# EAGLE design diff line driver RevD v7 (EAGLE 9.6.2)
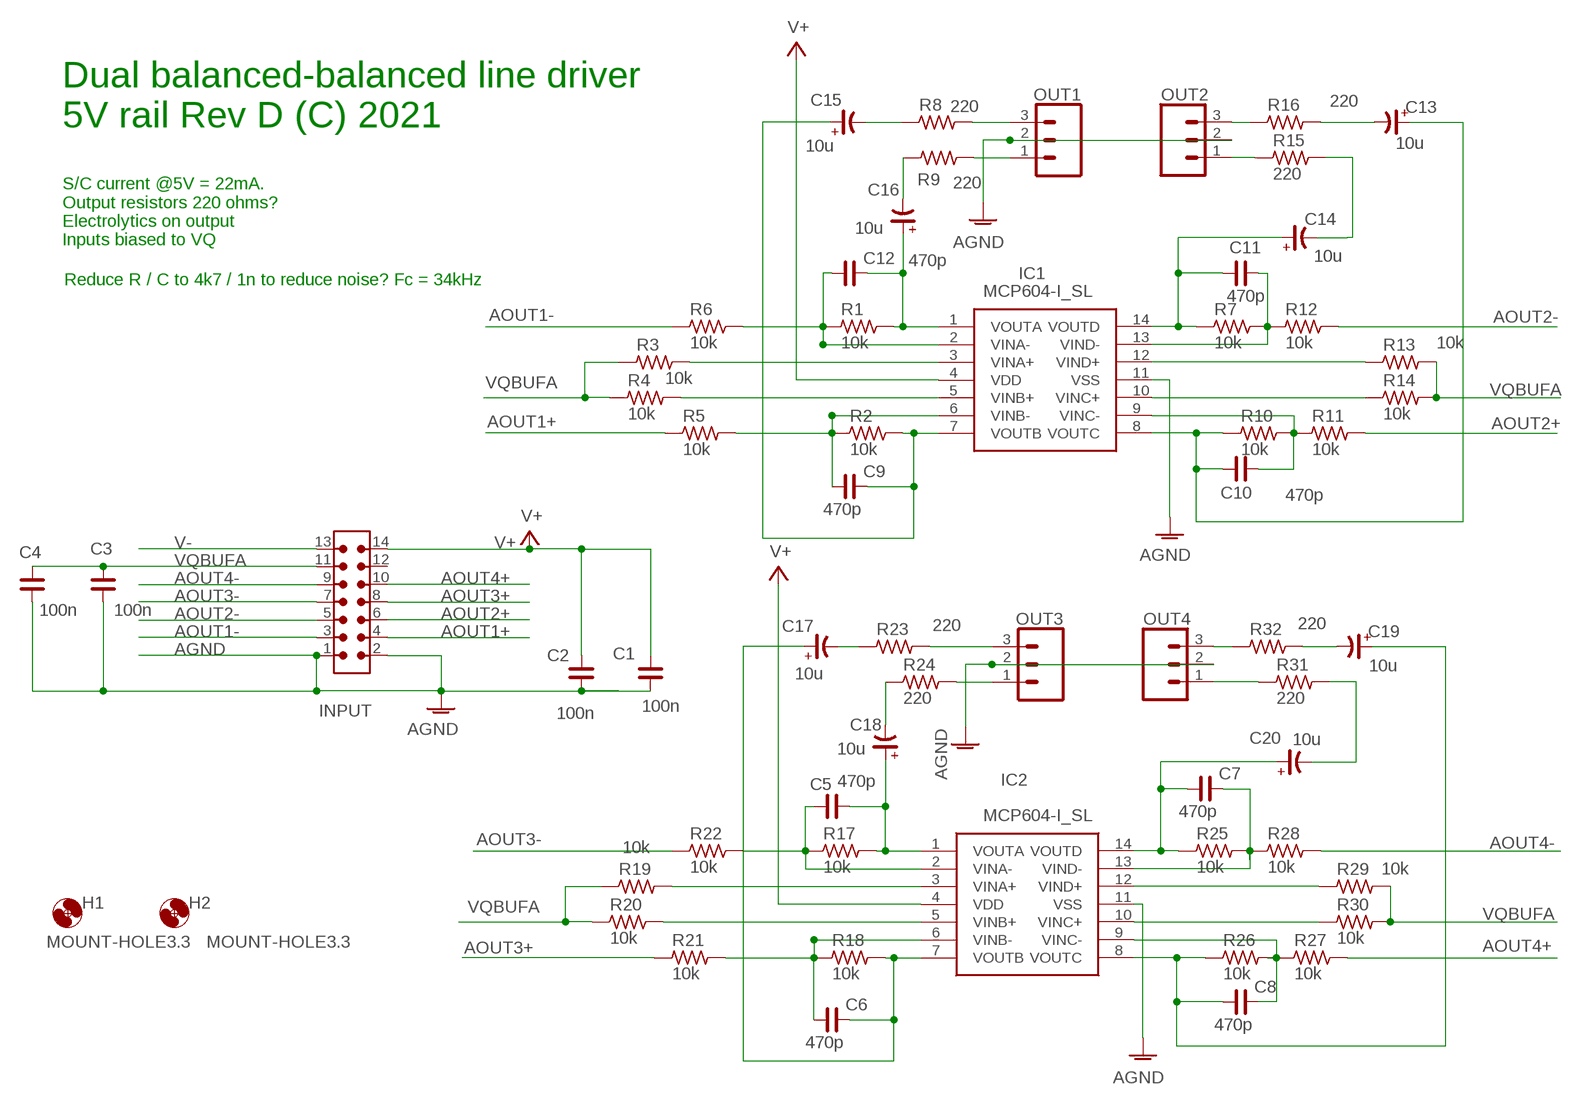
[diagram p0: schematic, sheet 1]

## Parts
C1  100n  C_0805  [C0805]
C2  100n  C_0805  [C0805]
C3  100n  C_0805  [C0805]
C4  100n  C_0805  [C0805]
C5  470p  C_0805  [C0805]
C6  470p  C_0805  [C0805]
C7  470p  C_0805  [C0805]
C8  470p  C_0805  [C0805]
C9  470p  C_0805  [C0805]
C10  470p  C_0805  [C0805]
C11  470p  C_0805  [C0805]
C12  470p  C_0805  [C0805]
C13  10u  CP_SV-C  [CSV-C]
C14  10u  CP_SV-C  [CSV-C]
C15  10u  CP_SV-C  [CSV-C]
C16  10u  CP_SV-C  [CSV-C]
C17  10u  CP_SV-C  [CSV-C]
C18  10u  CP_SV-C  [CSV-C]
C19  10u  CP_SV-C  [CSV-C]
C20  10u  CP_SV-C  [CSV-C]
H1  MOUNT-HOLE3.3  [3,3]
H2  MOUNT-HOLE3.3  [3,3]
IC1  MCP604-I_SL  [SOIC127P600X175-14N]
IC2  MCP604-I_SL  [SOIC127P600X175-14N]
INPUT  6120XX21621_61201421621  [61201421621]
OUT1  CONN_03  [1X03]
OUT2  CONN_03  [1X03]
OUT3  CONN_03  [1X03]
OUT4  CONN_03  [1X03]
R1  10k  R_0805  [R0805]
R2  10k  R_0805  [R0805]
R3  10k  R_0805  [R0805]
R4  10k  R_0805  [R0805]
R5  10k  R_0805  [R0805]
R6  10k  R_0805  [R0805]
R7  10k  R_0805  [R0805]
R8  220  R_0805  [R0805]
R9  220  R_0805  [R0805]
R10  10k  R_0805  [R0805]
R11  10k  R_0805  [R0805]
R12  10k  R_0805  [R0805]
R13  10k  R_0805  [R0805]
R14  10k  R_0805  [R0805]
R15  220  R_0805  [R0805]
R16  220  R_0805  [R0805]
R17  10k  R_0805  [R0805]
R18  10k  R_0805  [R0805]
R19  10k  R_0805  [R0805]
R20  10k  R_0805  [R0805]
R21  10k  R_0805  [R0805]
R22  10k  R_0805  [R0805]
R23  220  R_0805  [R0805]
R24  220  R_0805  [R0805]
R25  10k  R_0805  [R0805]
R26  10k  R_0805  [R0805]
R27  10k  R_0805  [R0805]
R28  10k  R_0805  [R0805]
R29  10k  R_0805  [R0805]
R30  10k  R_0805  [R0805]
R31  220  R_0805  [R0805]
R32  220  R_0805  [R0805]

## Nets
AGND: C1.1 C2.1 C3.1 C4.1 IC1.11(VSS) IC2.11(VSS) INPUT.1 INPUT.2 OUT1.2 OUT2.2 OUT3.2 OUT4.2
AOUT1+: INPUT.4 R5.1
AOUT1-: INPUT.3 R6.1
AOUT2+: INPUT.6 R11.2
AOUT2-: INPUT.5 R12.2
AOUT3+: INPUT.8 R21.1
AOUT3-: INPUT.7 R22.1
AOUT4+: INPUT.10 R27.2
AOUT4-: INPUT.9 R28.2
N$1: C12.1 IC1.2(VINA-) R1.1 R6.2
N$2: C11.1 C14.+ IC1.14(VOUTD) R7.1
N$3: IC1.3(VINA+) R3.2
N$4: C12.2 C16.+ IC1.1(VOUTA) R1.2
N$5: C9.2 C15.+ IC1.7(VOUTB) R2.2
N$6: IC1.5(VINB+) R4.2
N$7: C9.1 IC1.6(VINB-) R2.1 R5.2
N$8: C10.1 C13.+ IC1.8(VOUTC) R10.1
N$9: OUT2.3 R16.1
N$10: OUT2.1 R15.1
N$11: OUT1.3 R8.2
N$12: OUT1.1 R9.2
N$13: C5.2 C18.+ IC2.1(VOUTA) R17.2
N$14: C10.2 IC1.9(VINC-) R10.2 R11.1
N$15: C11.2 IC1.13(VIND-) R7.2 R12.1
N$16: IC1.12(VIND+) R13.1
N$17: IC1.10(VINC+) R14.1
N$19: C5.1 IC2.2(VINA-) R17.1 R22.2
N$20: IC2.3(VINA+) R19.2
N$21: IC2.5(VINB+) R20.2
N$22: C6.1 IC2.6(VINB-) R18.1 R21.2
N$23: OUT3.3 R23.2
N$24: OUT3.1 R24.2
N$25: C7.1 C20.+ IC2.14(VOUTD) R25.1
N$26: C8.1 C19.+ IC2.8(VOUTC) R26.1
N$27: OUT4.3 R32.1
N$28: OUT4.1 R31.1
N$29: C8.2 IC2.9(VINC-) R26.2 R27.1
N$30: C7.2 IC2.13(VIND-) R25.2 R28.1
N$31: IC2.12(VIND+) R29.1
N$32: IC2.10(VINC+) R30.1
N$33: C13.- R16.2
N$34: C14.- R15.2
N$35: C15.- R8.1
N$36: C18.- R24.1
N$37: C19.- R32.2
N$38: C20.- R31.2
N$39: C16.- R9.1
N$40: C17.- R23.1
N$41: C6.2 C17.+ IC2.7(VOUTB) R18.2
V+ [power]: C1.2 C2.2 IC1.4(VDD) IC2.4(VDD) INPUT.14
V- [power]: INPUT.13
VQBUFA: C3.2 C4.2 INPUT.11 R3.1 R4.1 R13.2 R14.2 R19.1 R20.1 R29.2 R30.2
Unconnected: INPUT.12

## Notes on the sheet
- Dual balanced-balanced line driver
  5V rail Rev D (C) 2021
- S/C current @5V = 22mA.
  Output resistors 220 ohms?
  Electrolytics on output
  Inputs biased to VQ
- Reduce R / C to 4k7 / 1n to reduce noise? Fc = 34kHz

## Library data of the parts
C1-C12 = rc-master-smd:C_: NON-POLARIZED CAP
C13-C20 = rc-master-smd:CP_: POLARIZED CAP
H1 H2 = holes:MOUNT-HOLE: MOUNTING HOLE with drill center marker
IC1 IC2 = SamacSys_Parts:MCP604-I_SL: MCP604-I/SL, Quad Operational Amplifier 2.8MHz CMOS, Rail-Rail, 3 V, 5 V, 14-Pin SOIC Source: Datasheet; DESCRIPTION: MCP604-I/SL, Quad Operational Amplifier 2.8MHz CMOS, Rail-Rail, 3 V, 5 V, 14-Pin SOIC; HEIGHT: 1.75mm; MANUFACTURER_NAME: Microchip; MANUFACTURER_PART_NUMBER: MCP604-I/SL; MOUSER_PART_NUMBER: 579-MCP604-I/SL; MOUSER_PRICE-STOCK: https://www.mouser.co.uk/ProductDetail/Microchip-Technology/MCP604-I-SL?qs=DYhulPWWrtuzz9AOJH%2FhgQ%3D%3D
INPUT = Wurth_Connectors_WR-BHD:6120XX21621_61201421621: WR-BHD 2.54 mm Male Box Header KIND PROPERTIES: Pitch 2.54 mm Gender:Male MATERIAL PROPERTIES: Insulator Material:PBT Insulator Flammability Rating UL94 V-0 Insulator Color:Black Contact Material :Copper Alloy Contact Plating :Gold Contact Type: Stamped GENERAL INFORMATION: Operating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; CONTACT-RESISTANCE: 20mOhm; DATASHEET-URL: https://katalog.we-online.com/em/datasheet/61201421621.pdf; GENDER: Male; IR: 3A; L: 25.44mm; MATES: WR-BHD 2.54mm Female IDC Connector with Strain Relief; MOUNT: THT; PACKAGING: Tray; PART-NUMBER: 61201421621; PINS: 14; PITCH: 2.54mm; TOL-R: max.; TYPE: Straight; WORKING-VOLTAGE: 250V(AC)
OUT1-OUT4 = SparkFun-Connectors:CONN_03: Multi connection point. Often used as Generic Header-pin footprint for 0.1 inch spaced/style header connections On any of the 0.1 inch spaced packages, you can populate with these: Break Away Headers - Straight (PRT-00116) Break Away Male Headers - Right Angle (PRT-00553) Female Headers (PRT-00115)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
R1-R32 = rc-master-smd:R_: RESISTOR

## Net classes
3 power: width 0.406 mm

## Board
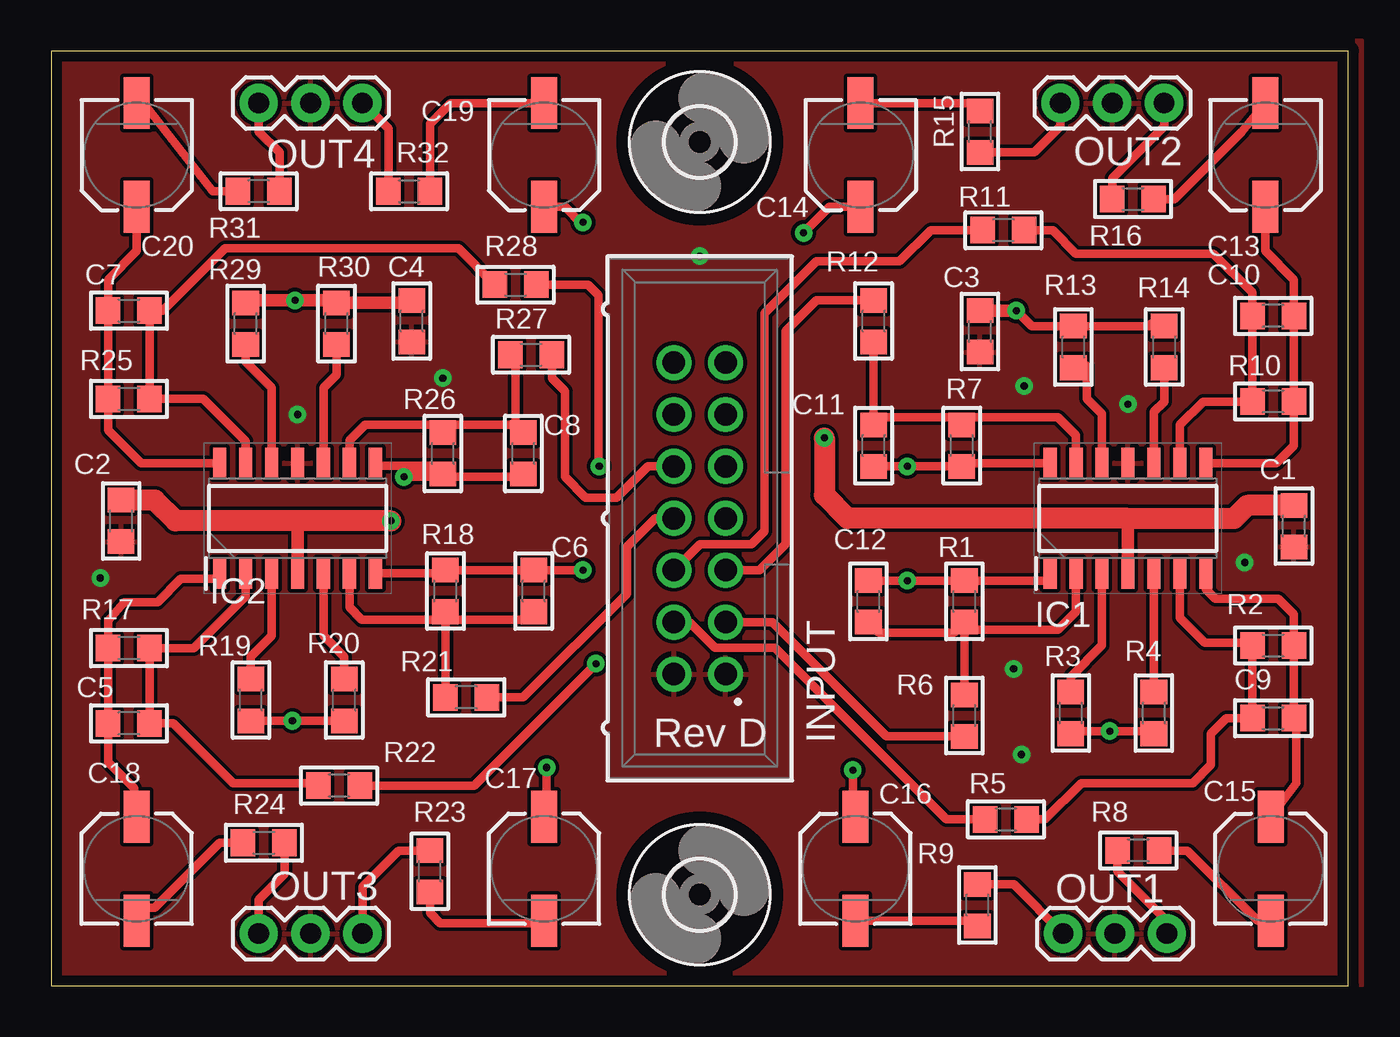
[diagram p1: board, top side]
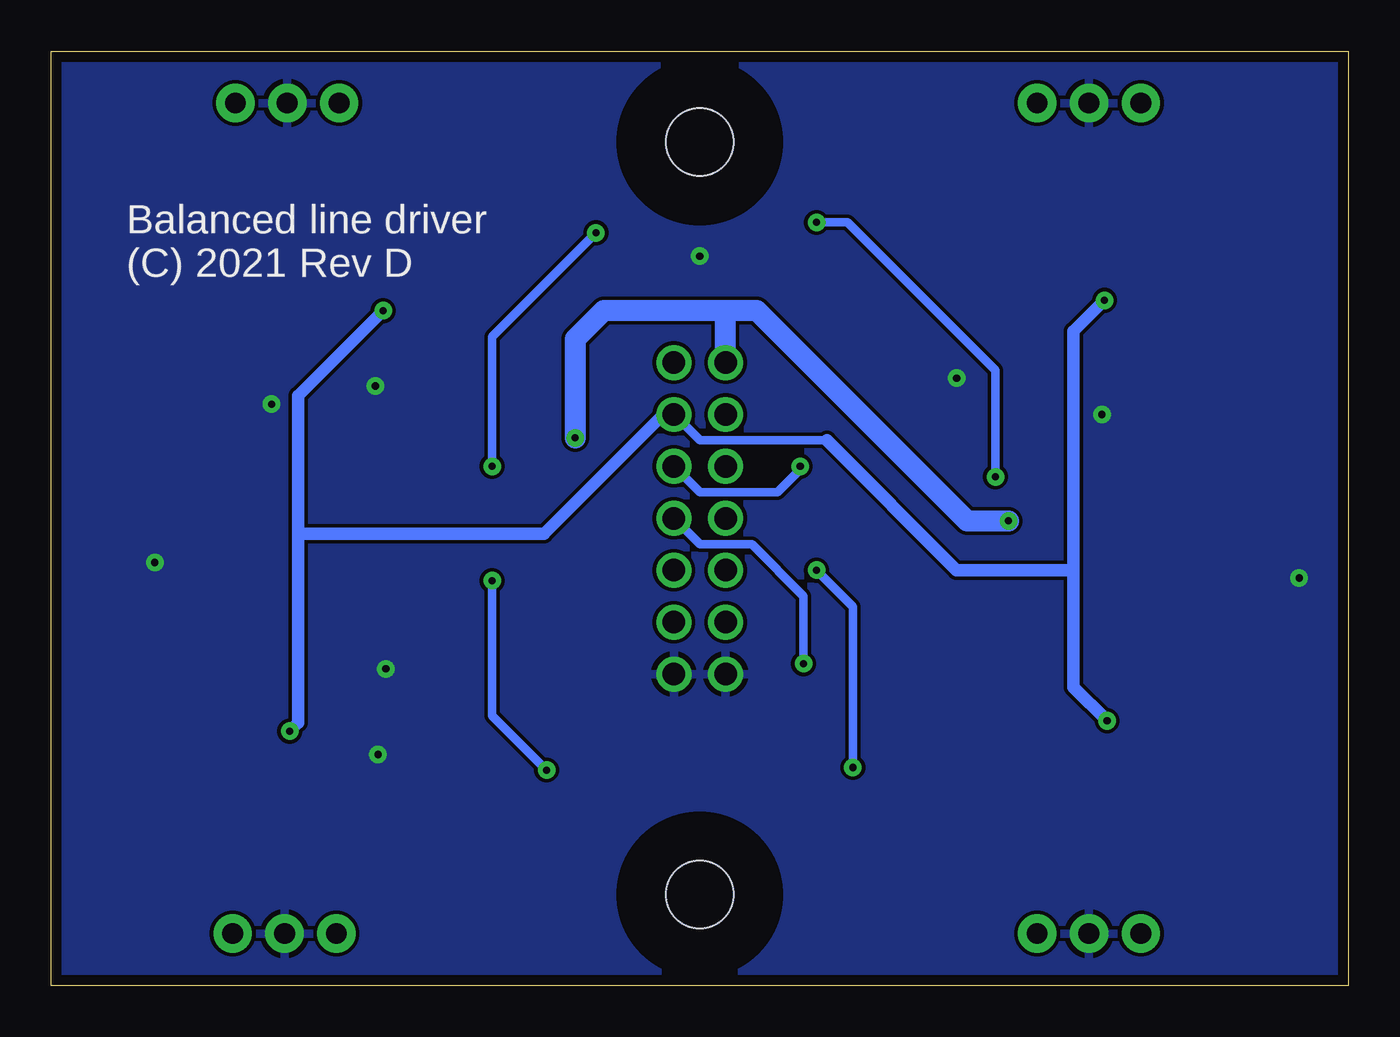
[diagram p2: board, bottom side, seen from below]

Size 63.5 x 45.72 mm. Coordinates in mm from the lower left corner, seen from the top.
Outline: 0,0 63.5,0 63.5,45.72 0,45.72 0,0
Copper layers (1*16): Top 0.035mm / dielectric 1.5mm / Bottom 0.035mm
Design rules "SparkFun - PCBWAY": minimum track width 8mil, minimum drill 13.5mil, track to track 7mil, track to pad 7mil, pad to pad 7mil, via to via 7mil, smd to smd 8mil, copper to edge 20mil, drill to drill 8mil, minimum pad ring 12mil, minimum via ring 10mil, stop-mask expansion 4mil, vias tented up to drill 25mil, thermal gap 10mil

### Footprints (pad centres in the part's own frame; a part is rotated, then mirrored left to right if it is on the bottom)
C0805 = smd 1.2 x 1.3: 1 -1.016,0; 2 1.016,0
CSV-C = smd 2.54 x 1.27: + -2.54,0; - 2.54,0
3,3 = hole 3.3: 0,0
SOIC127P600X175-14N = smd 1.5 x 0.65: 1 -2.7,3.81; 2 -2.7,2.54; 3 -2.7,1.27; 4 -2.7,0; 5 -2.7,-1.27; 6 -2.7,-2.54; 7 -2.7,-3.81; 8 2.7,-3.81; 9 2.7,-2.54; 10 2.7,-1.27; 11 2.7,0; 12 2.7,1.27; 13 2.7,2.54; 14 2.7,3.81
61201421621 = drill 1.1: 1 -7.62,-1.27; 2 -7.62,1.27; 3 -5.08,-1.27; 4 -5.08,1.27; 5 -2.54,-1.27; 6 -2.54,1.27; 7 0,-1.27; 8 0,1.27; 9 2.54,-1.27; 10 2.54,1.27; 11 5.08,-1.27; 12 5.08,1.27; 13 7.62,-1.27; 14 7.62,1.27
1X03 = drill 1.016 pad 1.88: 1 0,0; 2 2.54,0; 3 5.08,0
R0805 = smd 1.2 x 1.3: 1 -1.016,0; 2 1.016,0

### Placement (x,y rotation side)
C1  60.83,22.48 90 top
C2  3.43,22.73 90 top
C3  45.47,32 90 top
C4  17.65,32.51 90 top
C5  3.81,12.83 180 top
C6  23.62,19.3 90 top
C7  3.81,33.02 0 top
C8  23.11,26.04 90 top
C9  59.82,13.08 0 top
C10  59.82,32.77 180 top
C11  40.26,26.42 90 top
C12  40.01,18.8 90 top
C13  59.44,40.64 90 top
C14  39.62,40.64 90 top
C15  59.69,5.71 270 top
C16  39.37,5.71 270 top
C17  24.13,5.71 270 top
C18  4.19,5.71 270 top
C19  24.13,40.64 90 top
C20  4.19,40.64 90 top
H1  31.75,4.45 0 top
H2  31.75,41.28 0 top
IC1  52.7,22.86 90 top
IC2  12.06,22.86 90 top
INPUT  31.75,22.86 90 top
OUT1  49.53,2.54 0 top
OUT2  49.4,43.18 0 top
OUT3  10.16,2.54 0 top
OUT4  10.16,43.18 0 top
R1  44.7,18.8 90 top
R2  59.82,16.64 0 top
R3  49.91,13.34 90 top
R4  53.98,13.34 90 top
R5  46.74,8.13 0 top
R6  44.7,13.21 90 top
R7  44.58,26.42 90 top
R8  53.21,6.6 180 top
R9  45.34,3.94 90 top
R10  59.82,28.57 180 top
R11  46.61,36.96 180 top
R12  40.26,32.51 90 top
R13  50.04,31.24 90 top
R14  54.48,31.24 90 top
R15  45.47,41.78 90 top
R16  52.96,38.48 0 top
R17  3.81,16.51 180 top
R18  19.3,19.3 90 top
R19  9.78,13.97 90 top
R20  14.35,13.97 90 top
R21  20.32,14.1 180 top
R22  14.1,9.78 180 top
R23  18.54,5.59 90 top
R24  10.41,6.98 0 top
R25  3.81,28.7 0 top
R26  19.18,26.04 90 top
R27  23.5,30.86 0 top
R28  22.73,34.29 0 top
R29  9.53,32.38 90 top
R30  13.97,32.38 90 top
R31  10.16,38.86 180 top
R32  17.53,38.86 0 top

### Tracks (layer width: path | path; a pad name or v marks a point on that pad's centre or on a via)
AGND  (via drill 0.35)
  other vias: 52.7,28.45 12.06,27.94 2.41,19.94 58.42,20.7 47.12,15.49 19.18,29.72 47.5,11.3 47.62,29.34 31.75,35.69
  pour Bottom: -1.27,46.99 66.04,46.99 66.04,0 -1.27,0
  pour Top: -0.38,46.23 64.14,46.23 64.14,0 -0.38,0
AOUT1+
  Top 0.406: R5.1 43.81,8.13 35.42,16.52 32.5,16.52 31.24,17.78 INPUT.4
AOUT1-
  Top 0.406: R6.1 40.89,12.19 35.31,17.78 INPUT.3
AOUT2+
  Top 0.406: R11.2 43.05,36.96 41.53,35.43 37.47,35.43 34.92,32.89 34.92,22.22 34.29,21.59 31.75,21.59 INPUT.6
AOUT2-
  Top 0.406: R12.2 37.47,33.53 35.94,32 35.94,21.58 34.68,20.32 INPUT.5
AOUT3+
  Top 0.406: R21.1 23.11,14.1 28.19,19.18 28.19,21.46 29.59,22.86 INPUT.8
AOUT3-  (via drill 0.35)
  Top 0.406: R22.1 20.7,9.78 v26.67,15.75
  Bottom 0.406: INPUT.7 31.75,21.59 29.2,21.59 26.67,19.06 v26.67,15.75
AOUT4+
  Top 0.406: R27.2 24.51,29.72 25.15,29.08 25.15,24.89 26.16,23.88 27.69,23.88 29.21,25.4 INPUT.10
AOUT4-  (via drill 0.35)
  Top 0.406: R28.2 26.29,34.29 26.8,33.78 26.8,25.44 v26.83,25.4
  Bottom 0.406: INPUT.9 31.75,24.13 27.94,24.13 26.83,25.24 v26.83,25.4
N$1
  Top 0.406: R1.1 R6.2 | IC1.2 50.16,18.29 49.28,17.4 45.09,17.4 R1.1 | R1.1 44.2,17.27 40.51,17.27 C12.1
N$2  (via drill 0.35)
  Top 0.406: IC1.14 44.74,25.56 R7.1 v41.91,25.4 40.64,25.4 40.45,25.59 C11.1 | C14.+ 38.1,38.1 v36.83,36.83
  Bottom 0.406: v36.83,36.83 41.91,31.75 v41.91,25.4
N$3
  Top 0.406: R3.2 49.91,15.11 51.44,16.64 IC1.3
N$4  (via drill 0.35)
  Top 0.406: IC1.1 48.9,19.81 R1.2 v41.91,19.81 C12.2 | C16.+ 39.24,8.38 v39.24,10.54
  Bottom 0.406: v39.24,10.54 41.91,13.21 v41.91,19.81
N$5
  Top 0.406: IC1.7 56.52,19.4 56.99,18.92 60.07,18.92 60.83,18.16 R2.2 C9.2 60.96,12.95 60.96,9.91 C15.+
N$6
  Top 0.406: IC1.5 R4.2
N$7
  Top 0.406: IC1.6 55.24,18 56.48,16.76 58.67,16.76 R2.1 C9.1 57.53,13.08 56.77,12.32 56.77,10.79 55.88,9.91 50.42,9.91 48.64,8.13 R5.2
N$8
  Top 0.406: C13.+ 59.44,35.94 60.83,34.54 C10.1 R10.1 60.83,26.42 59.98,25.56 IC1.8
N$9
  Top 0.406: OUT2.3 54.48,42.04 51.94,39.5 R16.1
N$10
  Top 0.406: OUT2.1 49.4,42.04 48.13,40.77 R15.1
N$11
  Top 0.406: R8.2 52.2,5.59 54.61,3.17 OUT1.3
N$12
  Top 0.406: OUT1.1 47.12,4.95 R9.2
N$13
  Top 0.406: IC2.1 8,19.91 6.35,19.91 5.21,18.76 3.59,18.76 2.79,17.85 R17.2 C5.2 2.79,10.92 4.06,9.65 4.06,8.38 C18.+
N$14
  Top 0.406: R11.1 49.02,36.96 50.16,35.81 56.9,35.81 58.8,33.91 C10.2 R10.2 56.39,28.57 55.24,27.43 IC1.9
N$15
  Top 0.406: IC1.13 50.16,26.92 49.28,27.81 44.96,27.81 R7.2 44.2,27.81 40.64,27.81 C11.2 R12.1
N$16
  Top 0.406: R13.1 50.71,30.31 50.71,28.7 51.44,27.97 IC1.12
N$17
  Top 0.406: IC1.10 53.98,28.07 54.48,28.57 R14.1
N$19
  Top 0.406: IC2.2 9.53,19.05 6.99,16.51 R17.1 C5.1 5.97,12.83 8.91,9.88 13.03,9.89 R22.2
N$20
  Top 0.406: IC2.3 10.79,17.11 9.78,16.1 R19.2
N$21
  Top 0.406: R20.2 14.35,16.1 13.34,17.11 IC2.5
N$22
  Top 0.406: IC2.6 14.61,18.51 15.21,17.91 18.92,17.91 R18.1 | R18.1 R21.2 | C6.1 23.24,17.91 19.68,17.91 R18.1
N$23
  Top 0.406: R23.2 17.02,6.6 15.24,4.83 OUT3.3
N$24
  Top 0.406: OUT3.1 10.16,4.19 11.43,5.46 R24.2
N$25
  Top 0.406: IC2.14 4.41,25.56 2.79,27.18 R25.1 C7.1 2.79,34.54 4.19,35.94 C20.+
N$26  (via drill 0.35)
  Top 0.406: IC2.8 16,25.43 19.18,25.43 R26.1 17.4,25.02 v17.27,24.89 22.99,24.89 C8.1 | v26.04,37.34 25.97,37.28 25.15,38.1 C19.+
  Bottom 0.406: v26.04,37.34 24.51,37.34 17.27,30.1 v17.27,24.89
N$27
  Top 0.406: OUT4.3 16.51,41.91 R32.1
N$28
  Top 0.406: OUT4.1 10.16,41.78 11.18,40.77 R31.1
N$29
  Top 0.406: IC2.9 14.61,26.67 15.37,27.43 18.8,27.43 R26.2 19.56,27.43 22.73,27.43 | R27.1 22.73,30.61 22.73,27.43 | C8.2 22.73,27.43
N$30
  Top 0.406: IC2.13 9.53,26.63 7.45,28.7 R25.2 C7.2 5.46,33.02 8.51,36.07 19.94,36.07 R28.1
N$31
  Top 0.406: IC2.12 10.79,29.24 9.53,30.51 R29.1
N$32
  Top 0.406: R30.1 13.97,29.88 13.34,29.24 IC2.10
N$33
  Top 0.406: R16.2 54.99,38.48 58.29,41.78 C13.-
N$34
  Top 0.406: C14.- 45.47,43.18 R15.2
N$35
  Top 0.406: R8.1 55.63,6.6 59.05,3.17 C15.-
N$36
  Top 0.406: C18.- 4.06,3.81 5.08,3.81 8.26,6.98 R24.1
N$37
  Top 0.406: R32.2 18.54,42.16 19.56,43.18 C19.-
N$38
  Top 0.406: R31.2 7.91,38.86 4.53,43.18 C20.-
N$39
  Top 0.406: C16.- 44.8,3.17 R9.1
N$40
  Top 0.406: C17.- 23.98,3.05 19.05,3.05 18.54,3.56 R23.1
N$41  (via drill 0.35)
  Top 0.406: IC2.7 19.14,20.16 R18.2 C6.2 v26.04,20.32 | v24.26,10.67 24.26,8.39 C17.+
  Bottom 0.406: v26.04,20.32 24.26,18.54 v24.26,10.67
V+  (via drill 0.35)
  Top 0.406: v16.64,22.73 12.1,22.73
  Top 0.61: IC1.4 52.7,22.86 | 12.1,22.73 12.06,22.86 IC2.4
  Top 1.016: v37.85,26.8 37.85,24 38.99,22.86 52.7,22.86 57.91,22.86 58.55,23.49 C1.2 | v16.64,22.73 6.1,22.73 5.08,23.75 C2.2
  Bottom 1.016: 30.48,33.02 28.96,33.02 18.67,22.73 v16.64,22.73 | 30.48,33.02 36.45,33.02 37.85,31.62 v37.85,26.8 | INPUT.14 30.48,33.02
VQBUFA  (via drill 0.35)
  Top 0.406: R3.1 49.91,12.45 v51.82,12.45 53.95,12.45 R4.1 | v47.24,33.02 48.01,32.26 R13.2 53.72,32.26 53.88,32.41 54.32,32.42 R14.2 | 13.97,33.53 R30.2 | R19.1 v11.81,12.95 R20.1
  Top 0.61: R29.2 10.16,33.53 v11.94,33.53 13.97,33.53 | v47.24,33.02 C3.2 | R30.2 17.53,33.4 C4.2
  Bottom 0.406: INPUT.11 31.75,26.67 25.53,26.67
  Bottom 0.61: INPUT.11 33.53,27.94 39.37,22.1 51.41,22.1 | 51.41,22.1 51.41,12.86 v51.82,12.45 | 51.41,22.1 51.41,28.86 v47.24,33.02 | v11.94,33.53 13.46,32 13.46,20.32 | 25.53,26.67 19.18,20.32 13.46,20.32 | 13.46,20.32 13.46,14.61 v11.81,12.95

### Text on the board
tNames: Rev D
bNames: Balanced line driver / (C) 2021 Rev D

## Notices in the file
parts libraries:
rc-master-smd: Copyright (C) 2007, Bob Starr
SparkFun-Connectors: Licensing: Creative Commons ShareAlike 4.0 International - https://creativecommons.org/licenses/by-sa/4.0
Wurth_Connectors_WR-BHD: Copyright: Würth Elektronik
